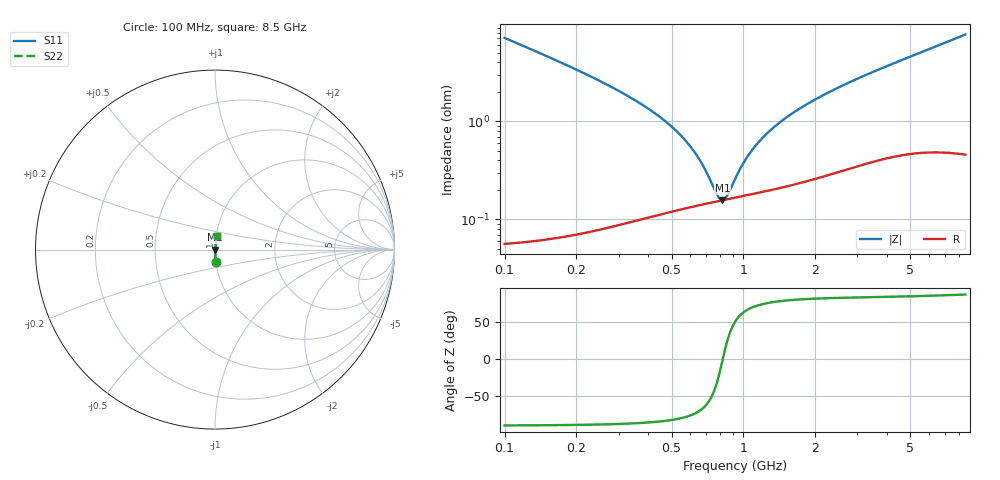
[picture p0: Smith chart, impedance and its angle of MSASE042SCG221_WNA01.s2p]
! MSASE042SCG221_WNA01  S-PARAMETER MODEL  ( General Type )
! Model Generated by TAIYO YUDEN Corporation (http://www.ty-top.com)
! Version 2.0
! TAIYO YUDEN Control No. 180301
! Copyright(c) 2016 TAIYO YUDEN CO.,LTD. All Rights Reserved.
! Product Description (link to TY-COMPAS)
! https://ds.yuden.co.jp/TYCOMPAS/or/detail?pn=MSASE042SCG221JWNA01&u=M
! Products Name : Multilayer Ceramic Capacitors
! Characteristics :
!  Capacitance : 220 pF , Rated Voltage : 16V , TCC : CG / C0G
!  Case Size : 0.4 x 0.2 / 0.016 x 0.008 [mm/inch] , Thickness : 0.2 / 0.008 [mm/inch]
!  (Conditions: Temperature = 25 degC , DC Bias Current/Voltage = 0A / 0V)
! External Node Assignments :
!  1  o---| |---o  2
! GND o---------o GND
! Frequency Range : 100MHz  -  8500MHz  [ 401 STEP ]
# MHz S RI R 50
! Freq[MHz].  S11 Real  S11 Imag  S21 Real  S21 Imag  S12 Real  S12 Imag  S22 Real  S22 Imag
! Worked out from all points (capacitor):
!   401 points, 100 MHz to 8.5 GHz, reference 50 ohm
!   read as one part in series: C = 222 pF near 102.2 MHz
!   lowest |Z| = 157 mohm at 815.9 MHz (marker M1)
!   series resonance near 819.7 MHz, so ESL is about 170 pH
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100  0.00554 -0.0704  0.9945 0.0704  0.9945 0.0704  0.00554 -0.0704
154.2121  0.00263 -0.0447  0.9974 0.0447  0.9974 0.0447  0.00263 -0.0447
222.4823  0.00162 -0.0296  0.9984 0.0296  0.9984 0.0296  0.00162 -0.0296
303.637  0.00128 -0.0201  0.9987 0.0201  0.9987 0.0201  0.00128 -0.0201
578.2564  0.00134 -0.00602  0.9987 0.00602  0.9987 0.00602  0.00134 -0.00602
668.0771  0.00142 -0.00347  0.9986 0.00347  0.9986 0.00347  0.00142 -0.00347
771.8496  0.00152 -0.00101  0.9985 0.00101  0.9985 0.00101  0.00152 -0.00101
798.0008  0.00155 -0.000449  0.9985 0.000449  0.9985 0.000449  0.00155 -0.000449
815.9254  0.00156 -7.73e-05  0.9984 7.73e-05  0.9984 7.73e-05  0.00156 -7.73e-05
852.9914  0.0016 0.000665  0.9984 -0.000665  0.9984 -0.000665  0.0016 0.000665
942.6632  0.00169 0.00233  0.9983 -0.00233  0.9983 -0.00233  0.00169 0.00233
996.4931  0.00174 0.00327  0.9983 -0.00327  0.9983 -0.00327  0.00174 0.00327
1101.251  0.00184 0.00496  0.9982 -0.00496  0.9982 -0.00496  0.00184 0.00496
1272.308  0.00202 0.00748  0.998 -0.00748  0.998 -0.00748  0.00202 0.00748
1502.954  0.00226 0.0106  0.9977 -0.0106  0.9977 -0.0106  0.00226 0.0106
1755.801  0.00255 0.0136  0.9974 -0.0136  0.9974 -0.0136  0.00255 0.0136
2074.094  0.00295 0.0173  0.9971 -0.0173  0.9971 -0.0173  0.00295 0.0173
2926.566  0.00408 0.026  0.9959 -0.026  0.9959 -0.026  0.00408 0.026
4317.005  0.00588 0.0389  0.9941 -0.0389  0.9941 -0.0389  0.00588 0.0389
5762.285  0.00745 0.0516  0.9926 -0.0516  0.9926 -0.0516  0.00745 0.0516
7116.102  0.00881 0.0634  0.9912 -0.0634  0.9912 -0.0634  0.00881 0.0634
8500  0.0103 0.0755  0.9897 -0.0755  0.9897 -0.0755  0.0103 0.0755
